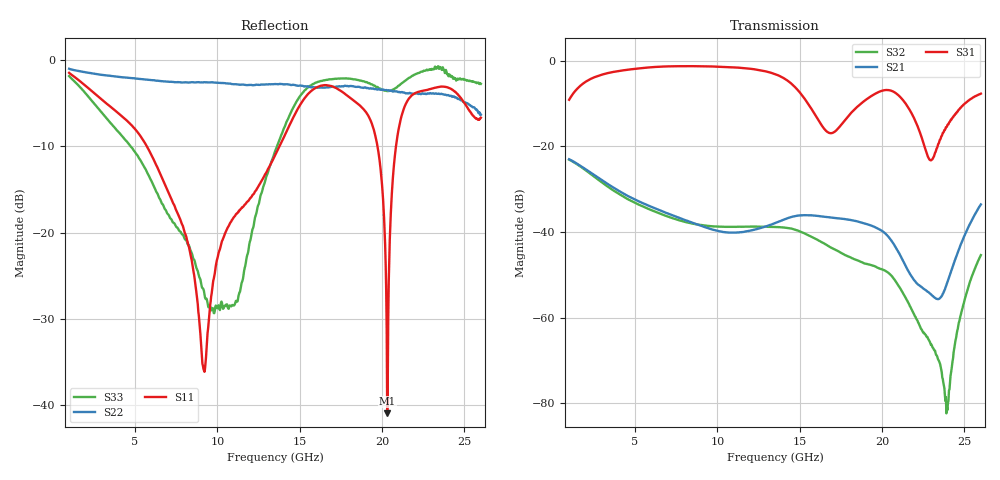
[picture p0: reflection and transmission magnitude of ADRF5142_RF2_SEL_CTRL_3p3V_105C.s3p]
! Device: ADRF5142
! Description: Silicon, SPDT Switch, Reflective
! Frequency: 8.00 GHz - 11.00 GHz
! Ports:
!  RFC = Port 1
!  RF1 = Port 2
!  RF2 = Port 3
! VDD = +3.3V
! VSS = -3.3V
! CTRL = +3.3V
! Temp = 85C
! Data:  Data was collected using an calibrated 4 port network analyzer.
!  The reference plane is the package pins of ADRF5142 switch.
! Notes: Analog Devices supplies this data as a sample of measured data
!  for this product.  Your particular data for this product may vary.
!  Data was taken at 85 degrees C.
!  Analog Devices reserves the right to change this data at anytime.
# HZ S DB R 50
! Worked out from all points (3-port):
!   801 points, 1 GHz to 26 GHz, reference 50 ohm
!   strongest paths, dB at 1 GHz, 7.25 GHz, 13.5 GHz, 19.75 GHz, 26 GHz:
!     S31: -9.1, -1.3, -3.1, -7.4, -7.7
!     S21: -23.0, -36.1, -37.9, -39.2, -33.6
!     S32: -23.1, -36.7, -38.8, -48.4, -45.4
!   lowest |S11| = -40.9 dB at 20.31 GHz (marker M1), VSWR 1.02, Z = 50.3 + j0.831 ohm
!   |S11| at or under -10 dB: 5.724 GHz to 13.77 GHz (8.045 GHz wide, 82.5 % of centre); 19.72 GHz to 20.84 GHz (1.12 GHz wide, 5.52 % of centre)
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1e9  -1.46 158.2  -23.00 -36.9  -9.10 35.3
     -23.00 -36.9  -0.99 170.9  -23.08 -54.7
     -9.10 35.3  -23.08 -54.7  -1.84 124.5
2.875e9  -4.38 130.1  -27.58 -85.0  -3.35 -17.6
         -27.58 -85.0  -1.67 157.2  -28.08 -136.4
         -3.35 -17.6  -28.08 -136.4  -5.85 36.1
5.7812e9  -10.21 97.5  -33.78 -124.0  -1.55 -86.5
          -33.78 -124.0  -2.26 141.3  -34.56 138.5
          -1.55 -86.5  -34.56 138.5  -13.18 -72.1
9.1875e9  -35.95 -57.5  -38.79 -156.2  -1.27 -163.6
          -38.79 -156.2  -2.55 119.3  -38.46 59.1
          -1.27 -163.6  -38.46 59.1  -26.77 -111.4
1.35e10  -11.06 -127.1  -37.93 -178.4  -3.09 87.3
         -37.93 -178.4  -2.76 94.1  -38.83 -47.4
         -3.09 87.3  -38.83 -47.4  -10.58 60.8
1.9e10  -5.95 84.2  -38.07 72.8  -9.15 53.4
        -38.07 72.8  -3.16 61.6  -47.42 133.7
        -9.15 53.4  -47.42 133.7  -2.54 -102.9
2.03125e10  -40.93 66.8  -40.78 39.9  -6.81 8.3
            -40.78 39.9  -3.49 52.7  -49.34 81.2
            -6.81 8.3  -49.34 81.2  -3.59 -114.2
2.11875e10  -6.43 -178.6  -46.10 24.7  -8.80 -30.0
            -46.10 24.7  -3.69 46.1  -53.73 41.3
            -8.80 -30.0  -53.73 41.3  -2.69 -120.2
2.39375e10  -3.13 59.1  -52.05 146.0  -15.39 15.9
            -52.05 146.0  -4.07 27.6  -81.01 -52.0
            -15.39 15.9  -81.01 -52.0  -1.61 -166.9
2.6e10  -6.66 -40.8  -33.55 136.2  -7.66 -31.5
        -33.55 136.2  -6.32 12.6  -45.40 142.3
        -7.66 -31.5  -45.40 142.3  -2.73 161.9
